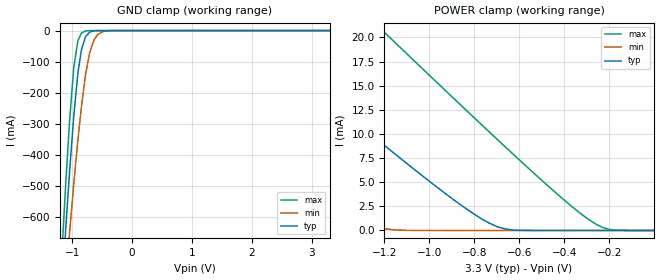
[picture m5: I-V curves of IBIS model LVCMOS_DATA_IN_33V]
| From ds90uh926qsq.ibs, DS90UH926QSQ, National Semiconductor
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[Model] LVCMOS_DATA_IN_33V
Model_type Input
Vinh = 2.0V
Vinl = 0.8V
C_comp   6.98pF   6.05pF   8.06pF
[Voltage Range]   3.3V   2.97V   3.63V
[Temperature Range]   25.0   130.0   -40.0
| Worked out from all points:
|   GND clamp passes 1 mA (typ) near -0.64 V on its own axis
|   POWER clamp passes 1 mA (typ) near -0.75 V on its own axis
[GND Clamp]
-3.3V     -7.729A    -6.4A      -8.836A
-1.171V   -833.9mA   -960.9mA   -719.2mA
-1.102V   -623.3mA   -790.6mA   -477.4mA
-1.043V   -454.3mA   -650.1mA   -290.9mA
-973.5mV  -277.4mA   -494.8mA   -119.9mA
-904.2mV  -136.9mA   -352.1mA   -32.52mA
-844.8mV  -61.18mA   -243.7mA   -7.904mA
-775.5mV  -19.33mA   -140.4mA   -1.013mA
-706.2mV  -4.959mA   -70.01mA   -78.98uA
-636.9mV  -979uA     -30.5mA    -10.61uA
-438.9mV  -5.524uA   -1.421mA   -493.3nA
3.293V    492.2nA    0A         630.2nA
[POWER Clamp]
-3.3V     49.92mA    32.15mA    67.97mA
-2.597V   36.03mA    20.71mA    52.03mA
-1.835V   21.06mA    8.532mA    34.8mA
-1.795V   20.29mA    7.916mA    33.91mA
-1.399V   12.62mA    2.095mA    25mA
-1.201V   8.841mA    190.7uA    20.57mA
-864.6mV  2.717mA    1.43uA     13.09mA
-696.3mV  373.5uA    1.191uA    9.393mA
-399.3mV  1.092uA    858nA      3.115mA
-260.7mV  851.6nA    730.9nA    661uA
-201.3mV  761.3nA    681.9nA    114.6uA
-3.3mV    503.4nA    542nA      1.401uA
